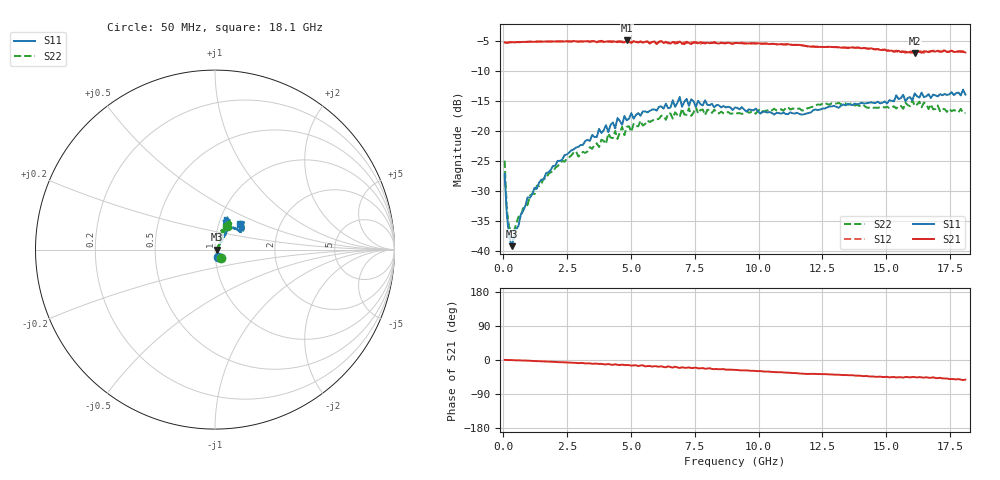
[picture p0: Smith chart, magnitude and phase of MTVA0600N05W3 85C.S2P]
! Network Analyzer HP8720D.06.14 Serial No. US36140669
!  8 Jul 2005  13:34:59
! Frequency  S11  S21  S12  S22
# HZ  S  DB R 50
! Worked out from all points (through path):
!   201 points, 50 MHz to 18.1 GHz, reference 50 ohm
!   highest |S21| = -4.85 dB at 4.833 GHz (marker M1); lowest = -6.9 dB at 16.11 GHz (marker M2)
!   group delay of S21, straight-line fit = 8.21 ps
!   lowest |S11| = -39.2 dB at 320.8 MHz (marker M3), VSWR 1.02, Z = 51.1 - j0.0499 ohm
!   |S11| at or under -10 dB: start of sweep to end of sweep
!   |S22| runs from -36.7 to -14.8 dB; largest |S21 - S12| = 0.026
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5e7  -27.15 -70.4  -5.16 0.3  -5.20 0.6  -24.92 -55.3
1.4025e8  -34.10 -53.5  -5.25 0.1  -5.23 0.0  -33.24 -47.1
2.305e8  -37.58 -28.8  -5.17 -0.1  -5.15 -0.2  -36.10 -29.1
3.2075e8  -39.19 -2.5  -5.12 -0.1  -5.15 -0.1  -36.41 -5.1
9.525e8  -31.02 44.8  -5.09 -1.8  -5.05 -1.9  -32.25 43.7
1.76475e9  -26.89 52.6  -5.01 -4.4  -5.02 -4.4  -27.13 51.6
3.1185e9  -22.28 57.0  -5.01 -7.9  -5.04 -8.3  -23.45 64.7
4.021e9  -18.98 60.1  -5.03 -11.6  -5.04 -10.7  -22.11 65.0
4.11125e9  -20.17 60.1  -4.99 -10.5  -5.07 -11.8  -20.37 65.3
4.47225e9  -17.78 56.8  -5.14 -12.6  -4.96 -11.9  -21.28 71.1
4.83325e9  -18.19 66.4  -4.85 -13.5  -5.06 -14.2  -19.26 61.7
6.09675e9  -15.93 63.6  -5.11 -17.7  -5.02 -17.7  -17.92 66.3
6.7285e9  -15.94 71.0  -5.16 -17.5  -5.40 -18.4  -16.85 62.5
6.909e9  -14.28 69.0  -5.03 -21.0  -5.12 -19.5  -17.63 62.0
6.99925e9  -15.92 68.9  -5.29 -19.2  -5.43 -21.0  -16.23 63.7
7.17975e9  -14.60 73.3  -5.05 -20.5  -5.29 -19.4  -17.25 59.3
7.54075e9  -15.94 65.9  -5.22 -19.9  -5.12 -22.6  -15.94 67.6
9.075e9  -16.03 69.3  -5.28 -26.1  -5.25 -26.2  -16.95 59.6
1.21435e10  -16.48 53.9  -5.88 -36.5  -5.83 -36.7  -15.88 60.3
1.512175e10  -14.83 35.8  -6.59 -45.8  -6.42 -45.4  -16.12 63.9
1.61145e10  -13.68 39.1  -6.92 -45.2  -6.63 -45.3  -15.77 65.8
1.81e10  -13.89 45.8  -6.85 -51.8  -7.03 -52.7  -16.95 63.3
